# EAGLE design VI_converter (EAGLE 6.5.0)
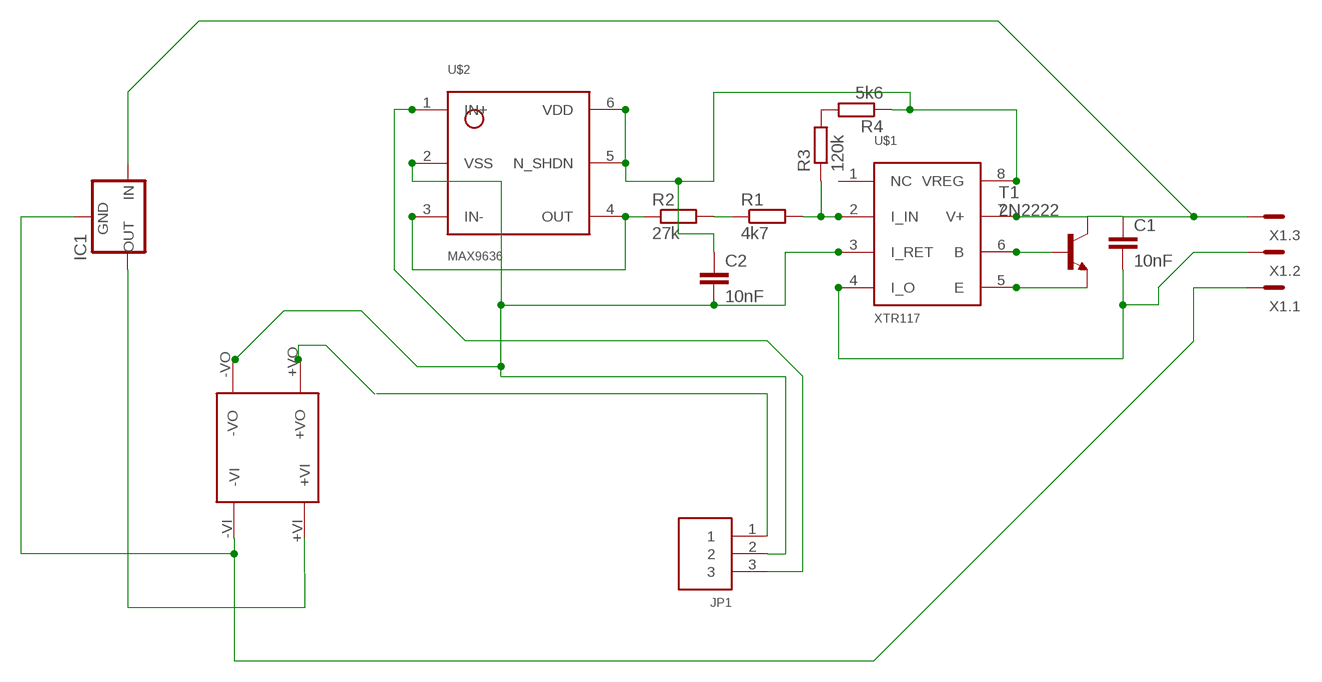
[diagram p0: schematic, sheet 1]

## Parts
C1  10nF  C-EUC1206  [C1206]
C2  10nF  C-EUC1206  [C1206]
IC1  78XXS  [78XXS]
JP1  3PIN  [B3B-PH-K-S]
R1  4k7  R-EU_M1206  [M1206]
R2  27k  R-EU_M1206  [M1206]
R3  120k  R-EU_M1206  [M1206]
R4  5k6  R-EU_M1206  [M1206]
T1  2N2222  [TO18]
U$1  XTR117  [MSOP8]
U$2  MAX9636  [SOT363]
U$3  ROE-0505S  [ROE-0505S]
X1  MC3  [MC3]

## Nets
GND: C2.2 JP1.2 U$1.3(I_RET) U$2.2(VSS)
N$1: T1.2(B) U$1.6(B)
N$2: T1.1(E) U$1.5(E)
N$3: C1.1 IC1.IN T1.3(C) U$1.7(V+) X1.3
N$4: R1.2 R3.1 U$1.2(I_IN)
N$5: R1.1 R2.2
N$6: R3.2 R4.2
N$7: C1.2 U$1.4(I_O) X1.2
N$8: R2.1 U$2.3(IN-) U$2.4(OUT)
N$9: JP1.3 U$2.1(IN+)
N$10: IC1.OUT U$3.+VI
N$11: IC1.GND U$3.-VI X1.1
N$12: JP1.1
VDD: C2.1 R4.1 U$1.8(VREG) U$2.5(N_SHDN) U$2.6(VDD)
Unconnected: U$1.1(NC) U$3.+VO U$3.-VO

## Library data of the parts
C1 C2 = resistor:C-EU: CAPACITOR, European symbol
IC1 = v-reg:78XXS: VOLTAGE REGULATOR
JP1 = jst_eph:3PIN
R1-R4 = resistor:R-EU_: RESISTOR, European symbol
T1 = transistor:2N2222: NPN TRANSISTOR
U$1 = rpascoal:XTR117
U$2 = rpascoal:MAX9636
U$3 = carpintas:ROE-0505S: ROE-0505S from RECOM Power
X1 = con-phoenix-381_l:MC3: Mini-Combicon 3.81mm horizontal 3-polig (ohne Gegenstecker)

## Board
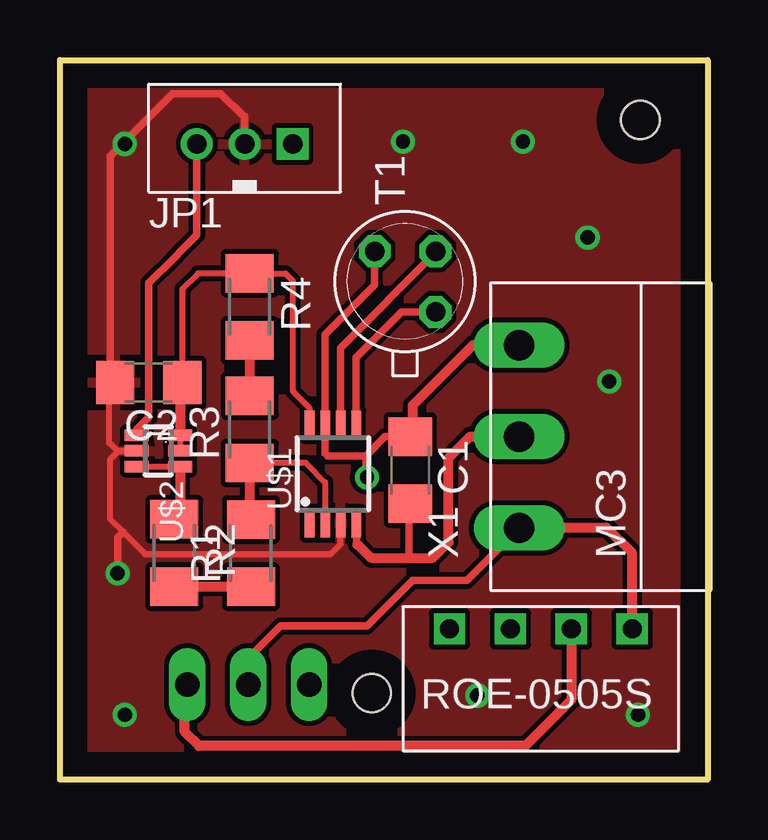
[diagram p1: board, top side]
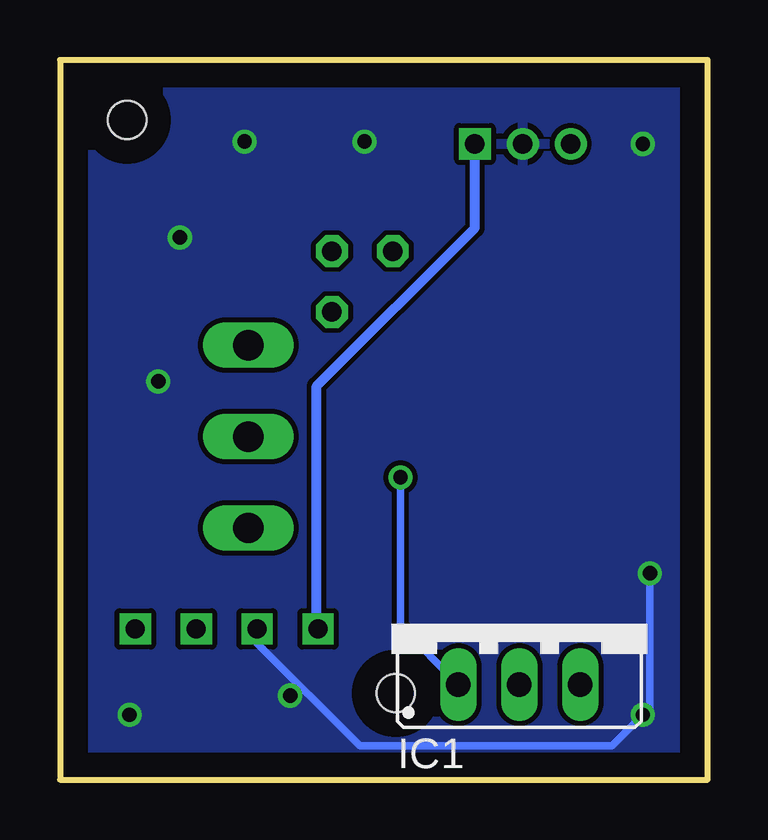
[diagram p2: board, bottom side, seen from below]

Size 27 x 30 mm. Coordinates in mm from the lower left corner, seen from the top.
Outline: 0,30 27,30 27,0 0,0 0,30
Copper layers (1*16): Top 0.035mm / dielectric 1.5mm / Bottom 0.035mm
Design rules "default *": minimum track width 8mil, minimum drill 20mil, track to track 8mil, track to pad 8mil, pad to pad 8mil, via to via 8mil, smd to smd 8mil, copper to edge 40mil, drill to drill 8mil, minimum pad ring 10mil, minimum via ring 8mil, stop-mask expansion 4mil, vias tented up to drill 0mil, thermal gap 10mil
Holes 1.6 mm at 24.2,27.5 13,3.6

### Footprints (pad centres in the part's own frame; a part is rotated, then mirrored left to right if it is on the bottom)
C1206 = smd 1.6 x 1.8: 1 -1.4,0; 2 1.4,0
78XXS = drill 1.016 long: GND 0,-2.54; IN -2.54,-2.54; OUT 2.54,-2.54
B3B-PH-K-S = drill 0.813 square: 1 2,0 | drill 0.813: 2 0,0; 3 -2,0
M1206 = smd 1.6 x 2: 1 -1.4,0; 2 1.4,0
TO18 = drill 0.813 octagon: 1 -1.27,-1.27; 2 1.27,-1.27; 3 1.27,1.27
MSOP8 = smd 0.4 x 1.2: 1 -0.975,-2.05; 2 -0.325,-2.05; 3 0.325,-2.05; 4 0.975,-2.05; 5 0.975,2.05; 6 0.325,2.05; 7 -0.325,2.05; 8 -0.975,2.05
SOT363 = smd 0.48 x 1: 1 -0.65,-0.65; 2 0,-0.65; 3 0.65,-0.65; 4 0.65,1.15; 5 0,1.15; 6 -0.65,1.15
ROE-0505S = drill 0.8 square: +VI 4.48,0.92; +VO 9.56,0.92; -VI 1.94,0.92; -VO 7.02,0.92
MC3 = drill 1.27 long: 1 -3.81,0; 2 0,0; 3 3.81,0

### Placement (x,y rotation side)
C1  14.6,12.9 270 top
C2  3.7,16.55 180 top
IC1  7.85,6.5 0 bottom
JP1  7.7,26.5 0 top
R1  7.96,9.44 90 top
R2  4.77,9.45 270 top
R3  7.91,14.6 90 top
R4  7.91,19.71 270 top
T1  14.39,20.76 90 top
U$1  11.38,12.74 0 top
U$2  3.85,13.7 270 top
U$3  25.8,7.2 180 top
X1  19.15,14.3 90 top

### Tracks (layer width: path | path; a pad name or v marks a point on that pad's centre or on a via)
GND  (via drill 0.6)
  Top 0.254: U$1.3 11.71,9.8 11.3,9.4 3.55,9.4 2.62,10.32 2.1,10.85 2.1,13.35 2.45,13.7 U$2.2 2.4,13.7 2.05,14.05 2.05,16.3 C2.2
  Top 0.305: v2.4,8.6 2.4,10.1 2.62,10.32 | C2.2 2.1,16.75 2.1,26 4.7,28.6 6.7,28.6 7.65,27.65 7.7,27.65 JP1.2
  Bottom 0.305: 18.78,5.68 14.5,1.4 4,1.4 v2.7,2.7 2.4,3 v2.4,8.6
  other vias: 2.7,26.5 14.3,26.6 19.3,26.6 22,22.6 22.9,16.6 24.1,2.7 17.4,3.5
  pour Bottom: -0.3,30.5 26.8,30.5 26.8,-0.4 -0.4,-0.4 -0.4,30.6
  pour Top: -0.5,30.7 27.3,30.7 27.3,-0.9 -0.5,-0.9 -0.5,30.6
N$1
  Top 0.254: T1.2 15.66,21.96 | U$1.6
  Top 0.305: 15.66,21.96 11.7,18 U$1.6
N$2
  Top 0.305: T1.1 14.24,19.49 12.35,17.6 U$1.5
N$3  (via drill 0.6)
  Top 0.254: 11.15,13.5 11.05,13.6
  Top 0.305: 11.05,13.6 U$1.7 11.05,18.55 13.12,20.62 T1.3 | 12.75,13.5 11.15,13.5 | 12.75,13.5 13.55,14.3 C1.1 | v12.8,12.6 12.75,12.65 12.75,13.5
  Top 0.406: X1.3 17.21,18.11 14.7,15.6 14.7,14.4 C1.1
  Bottom 0.305: IC1.IN 12.8,6.4 v12.8,12.6
N$4
  Top 0.254: U$1.2 11.05,12.39 10.25,13.2 R3.1 | 7.91,10.89 R1.2
  Top 0.406: R3.1 7.91,10.89
N$5
  Top 0.254: R1.1
  Top 0.406: R2.2 R1.1
N$6
  Top 0.406: R4.2 R3.2
N$7
  Top 0.305: C1.2 14.55,11.5 14.55,9.24 | 12.4,9.8 12.36,9.8 U$1.4
  Top 0.406: 12.4,9.8 12.96,9.24 14.55,9.24 15.54,9.24 16.2,9.9 16.2,13.4 17.1,14.3 X1.2
N$8
  Top 0.254: 5,11.08 R2.1 | U$2.3 U$2.4
  Top 0.406: U$2.4 5,11.08
N$9
  Top 0.305: U$2.1 3.2,14.6 3.7,15.1 3.7,20.7 4.75,21.75 5.11,22.11 5.7,22.7 JP1.3
N$10
  Top 0.406: U$3.+VI 21.32,3.32 19.4,1.4 5.8,1.4 5.2,2 5.2,3.88 IC1.OUT
N$11
  Top 0.305: IC1.GND 7.85,5.05 9.2,6.4 12.8,6.4 14.7,8.3 16.96,8.3 X1.1
  Top 0.406: U$3.-VI 23.86,9.44 22.8,10.5 X1.1
N$12
  Bottom 0.406: 16.3,6.34 16.3,16.4 9.7,23 JP1.1
VDD
  Top 0.254: U$2.6 U$2.5 | 5,16.45 C2.1 5.1,20.45 5.75,21.1 R4.1 9.4,21.1 9.7,20.8 9.7,16.2 10.4,15.49 U$1.8
  Top 0.406: 5,16.45 U$2.6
